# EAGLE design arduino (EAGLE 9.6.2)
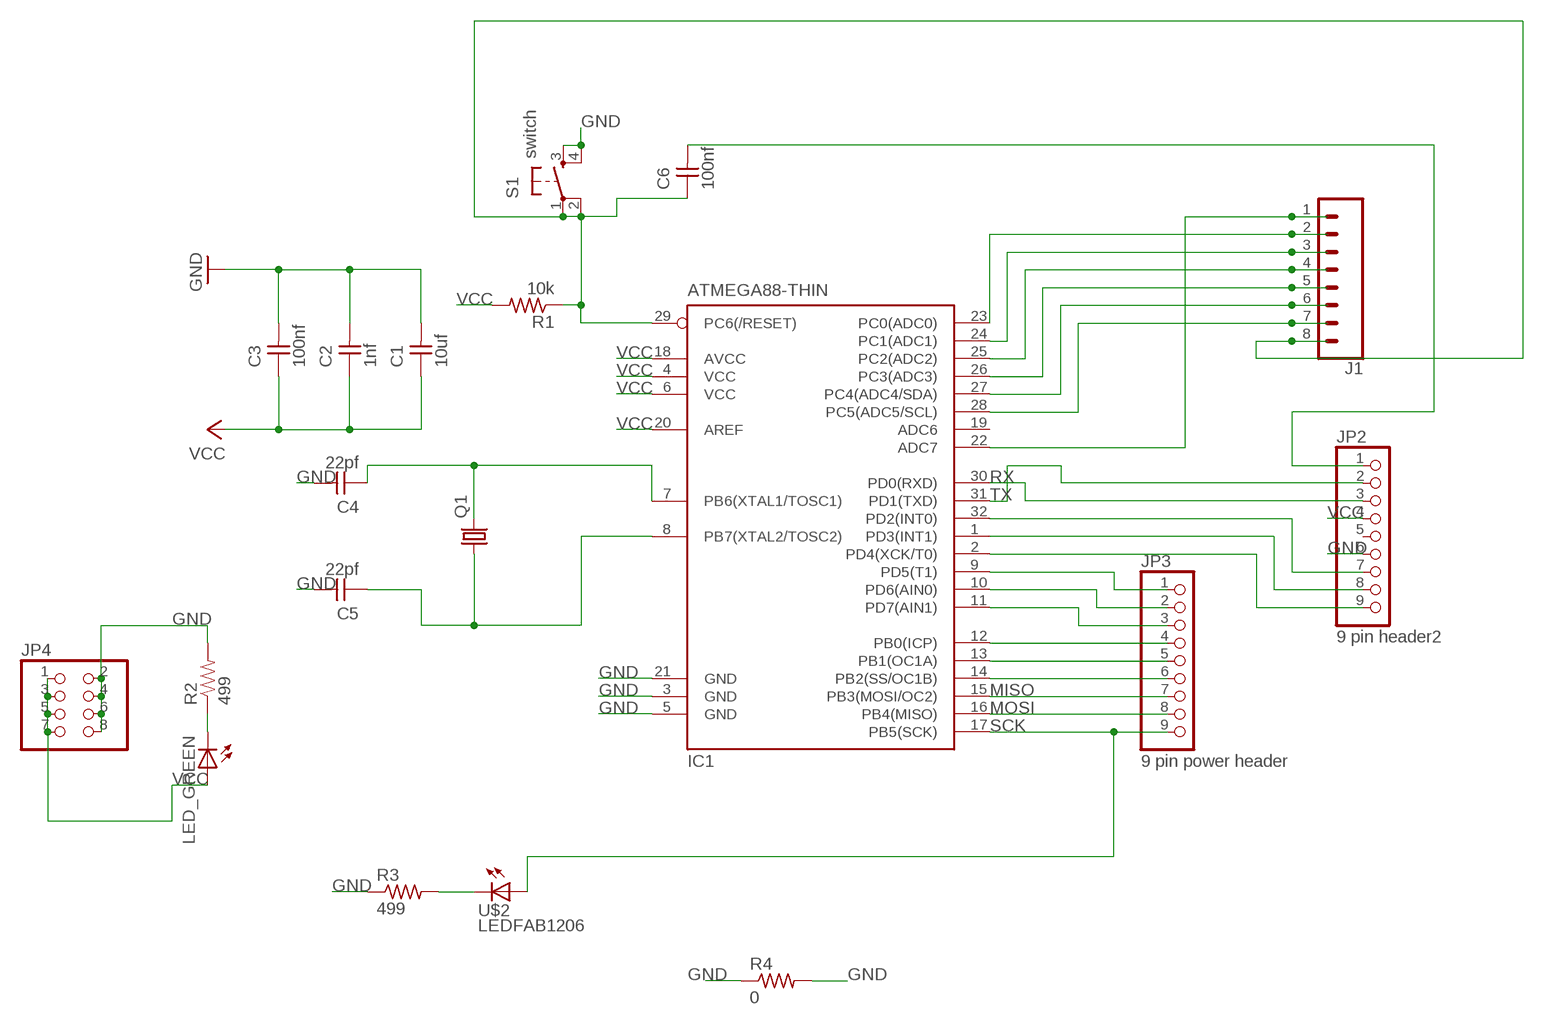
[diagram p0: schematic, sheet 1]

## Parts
C1  10uf  CAP-UNPOLARIZEDFAB  [C1206FAB]
C2  1nf  CAP-UNPOLARIZEDFAB  [C1206FAB]
C3  100nf  CAP-UNPOLARIZEDFAB  [C1206FAB]
C4  22pf  CAP-UNPOLARIZEDFAB  [C1206FAB]
C5  22pf  CAP-UNPOLARIZEDFAB  [C1206FAB]
C6  100nf  CAP-UNPOLARIZEDFAB  [C1206FAB]
IC1  ATMEGA88-THIN  [TQFP32-08THIN]
J1  CONN_08LONGPADS  [1X08_LONGPADS]
JP2  9 pin header2  PINHD-1X9  [1X09]
JP3  9 pin power header  PINHD-1X9  [1X09]
JP4  PINHD-2X4  [2X04]
LED_GREEN  LED1206  [1206]
Q1  CRYSTALHC49S  [HC49/S]
R1  10k  RES-US1206FAB  [R1206FAB]
R2  499  RESISTOR1206  [1206]
R3  499  RES-US1206FAB  [R1206FAB]
R4  0  RES-US1206FAB  [R1206FAB]
S1  switch  6MM_SWITCH6MM_SWITCH  [6MM_SWITCH]
U$2  LEDFAB1206  [LED1206FAB]

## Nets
GND: C1.2 C2.2 C3.2 C4.2 C5.2 IC1.3(GND) IC1.5(GND) IC1.21(GND) JP2.6 JP4.2 JP4.4 JP4.6 JP4.8 R2.2 R3.1 R4.1 R4.2 S1.3(S) S1.4(S1)
MISO: IC1.15(PB3(MOSI/OC2)) JP3.7
MOSI: IC1.16(PB4(MISO)) JP3.8
N$1: IC1.23(PC0(ADC0)) J1.2
N$2: IC1.24(PC1(ADC1)) J1.3
N$3: IC1.25(PC2(ADC2)) J1.4
N$4: IC1.26(PC3(ADC3)) J1.5
N$5: IC1.27(PC4(ADC4/SDA)) J1.6
N$6: IC1.28(PC5(ADC5/SCL)) J1.7
N$7: C6.2 JP2.1
N$8: C6.1 IC1.29(PC6(/RESET)) J1.8 R1.1 S1.1(P) S1.2(P1)
N$9: IC1.22(ADC7) J1.1
N$11: IC1.2(PD4(XCK/T0)) JP2.9
N$12: IC1.1(PD3(INT1)) JP2.8
N$13: IC1.32(PD2(INT0)) JP2.7
N$16: IC1.9(PD5(T1)) JP3.1
N$17: IC1.10(PD6(AIN0)) JP3.2
N$18: IC1.11(PD7(AIN1)) JP3.3
N$19: IC1.12(PB0(ICP)) JP3.4
N$20: IC1.13(PB1(OC1A)) JP3.5
N$21: IC1.14(PB2(SS/OC1B)) JP3.6
N$23: LED_GREEN.2(C) R2.1
N$26: R3.2 U$2.2(C)
N$30: C4.1 IC1.7(PB6(XTAL1/TOSC1)) Q1.2
N$31: C5.1 IC1.8(PB7(XTAL2/TOSC2)) Q1.1
RX: IC1.30(PD0(RXD)) JP2.3
SCK: IC1.17(PB5(SCK)) JP3.9 U$2.1(A)
TX: IC1.31(PD1(TXD)) JP2.2
VCC: C1.1 C2.1 C3.1 IC1.4(VCC) IC1.6(VCC) IC1.18(AVCC) IC1.20(AREF) JP2.4 JP4.1 JP4.3 JP4.5 JP4.7 LED_GREEN.1(A) R1.2
Unconnected: IC1.19(ADC6) JP2.5

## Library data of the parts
C1-C6 = fab:CAP-UNPOLARIZED
IC1 = fab:ATMEGA88-THIN
J1 = SparkFun-Connectors:CONN_08: Multi connection point. Often used as Generic Header-pin footprint for 0.1 inch spaced/style header connections On any of the 0.1 inch spaced packages, you can populate with these: Break Away Headers - Straight (PRT-00116) Break Away Male Headers - Right Angle (PRT-00553) Female Headers (PRT-00115)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
JP2 JP3 = pinhead:PINHD-1X9: PIN HEADER
JP4 = pinhead:PINHD-2X4: PIN HEADER
LED_GREEN = 01_FAB_Hello:LED
Q1 = crystal:CRYSTAL: CRYSTAL; OC_FARNELL: 1667008; OC_NEWARK: unknown
R1 R3 R4 = fab:RES-US: Resistor (US Symbol)
R2 = 01_SparkFun:RESISTOR: Resistor
S1 = fab:6MM_SWITCH: OMRON SWITCH
U$2 = fab:LED: LED

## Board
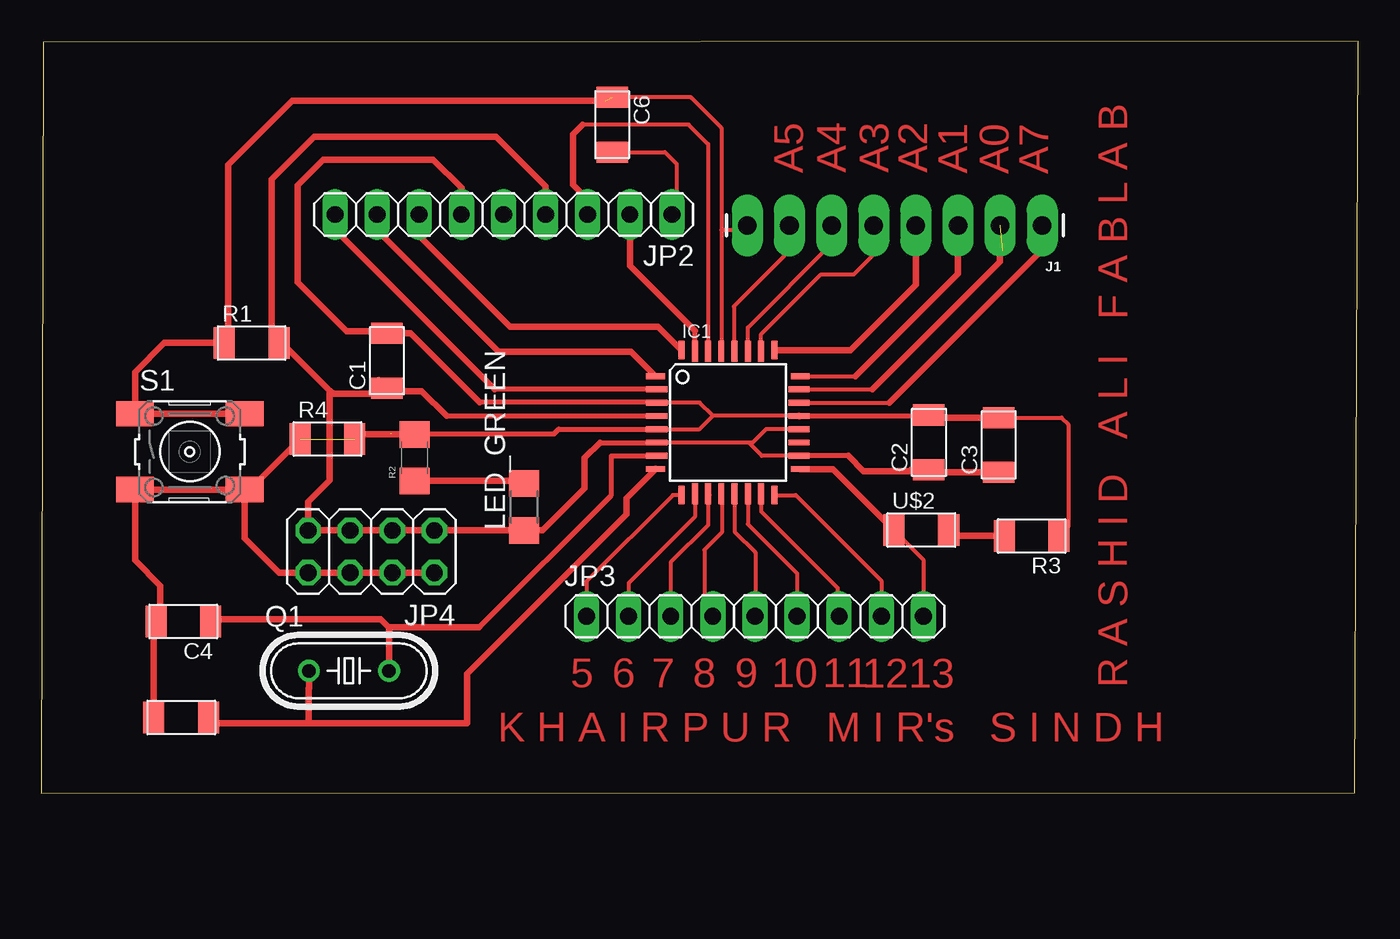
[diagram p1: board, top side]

Size 79.4 x 45.33 mm. Coordinates in mm from the lower left corner, seen from the top.
Outline: 0,0 79.2,0.02 79.4,45.33 0.1,45.28 0,0
Copper layers (1*16): Top 0.035mm / dielectric 1.5mm / Bottom 0.035mm
Design rules "default *": minimum track width 10mil, minimum drill 24mm, track to track 8mil, track to pad 8mil, pad to pad 8mil, via to via 8mil, smd to smd 8mil, copper to edge 40mil, drill to drill 8mil, minimum pad ring 10mil, minimum via ring 8mil, stop-mask expansion 4mil, vias tented up to drill 0mil, thermal gap 10mil

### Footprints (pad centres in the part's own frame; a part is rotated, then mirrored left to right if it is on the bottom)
C1206FAB = smd 1.27 x 1.905: 1 -1.651,0; 2 1.651,0
TQFP32-08THIN = smd 1.118 x 0.356: 1 -4.369,2.8; 8 -4.369,-2.8; 17 4.369,-2.8; 24 4.369,2.8 | smd 1.27 x 0.356: 2 -4.293,2; 3 -4.293,1.2; 4 -4.293,0.4; 5 -4.293,-0.4; 6 -4.293,-1.2; 7 -4.293,-2; 18 4.293,-2; 19 4.293,-1.2; 20 4.293,-0.4; 21 4.293,0.4; 22 4.293,1.2; 23 4.293,2 | smd 0.356 x 1.118: 9 -2.8,-4.369; 16 2.8,-4.369; 25 2.8,4.369; 32 -2.8,4.369 | smd 0.356 x 1.27: 10 -2,-4.293; 14 1.2,-4.293; 15 2,-4.293; 26 2,4.293; 27 1.2,4.293; 31 -2,4.293 | smd 0.35 x 1.27: 11 -1.2,-4.293; 12 -0.4,-4.293; 13 0.4,-4.293; 28 0.4,4.293; 29 -0.4,4.293; 30 -1.2,4.293
1X08_LONGPADS = drill 1.118 pad 1.88 long: 1 0,0; 2 2.54,0; 3 5.08,0; 4 7.62,0; 5 10.16,0; 6 12.7,0; 7 15.24,0; 8 17.78,0
1X09 = drill 1.016 long: 1 -10.16,0; 2 -7.62,0; 3 -5.08,0; 4 -2.54,0; 5 0,0; 6 2.54,0; 7 5.08,0; 8 7.62,0; 9 10.16,0
2X04 = drill 1.016 octagon: 1 -3.81,-1.27; 2 -3.81,1.27; 3 -1.27,-1.27; 4 -1.27,1.27; 5 1.27,-1.27; 6 1.27,1.27; 7 3.81,-1.27; 8 3.81,1.27
1206 = smd 1.6 x 1.803: 1 -1.422,0; 2 1.422,0
HC49/S = drill 0.813: 1 -2.413,0; 2 2.413,0
R1206FAB = smd 1.27 x 1.905: 1 -1.651,0; 2 1.651,0
1206' = smd 1.6 x 1.8: 1 -1.4,0; 2 1.4,0
6MM_SWITCH = smd 2.286 x 1.524: 1 -3.302,2.286; 2 3.302,2.286; 3 -3.302,-2.286; 4 3.302,-2.286
LED1206FAB = smd 1.27 x 1.905: 1 -1.651,0; 2 1.651,0

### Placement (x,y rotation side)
C1  20.83,26.09 90 top
C2  53.52,21.16 90 top
C3  57.73,21.01 90 top
C4  8.56,10.36 180 top
C5  8.43,4.57 180 top
C6  34.42,40.31 270 top
IC1  41.4,22.35 0 top
J1  60.35,34.24 180 top
JP2  27.86,34.9 180 top
JP3  43.03,10.67 0 top
JP4  19.89,14.58 180 top
LED_GREEN  29.11,17.27 90 top
Q1  18.54,7.39 0 top
R1  12.67,27.15 0 top
R2  499  [1206']  22.5,20.24 90 top
R3  59.72,15.52 180 top
R4  17.25,21.36 0 top
S1  8.94,20.6 0 top
U$2  53.06,15.87 0 top

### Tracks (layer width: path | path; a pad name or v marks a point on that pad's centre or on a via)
GND  (2 unrouted)
  Top 0.254: IC1.21 40.49,22.75 | IC1.3 39.69,23.55 40.49,22.75 | 40.49,22.75 39.69,21.95 IC1.5 | C3.2 61.52,22.66 61.92,22.25 61.92,16.08 R3.1
  Top 0.305: 26.43,23.58 37.08,23.58 IC1.3 | 21.08,21.67 30.91,21.67 31.2,21.95 IC1.5 | IC1.21 53.46,22.75 C2.2
  Top 0.406: 45.71,22.73 IC1.21 | C3.2 53.67,22.66 C2.2 | 7.19,4.17 C5.2 6.78,10.24 C4.2 | C4.2 6.91,10.82 | 26.43,23.58 22.28,27.74 C1.2 20.7,27.86 18.39,27.86 15.44,30.81 15.44,36.65 16.99,38.2 23.62,38.2 25.32,36.5 JP2.6 | S1.4 S1.3 5.64,14.05 7.16,12.52 7.16,10.62 C4.2 | JP4.2 JP4.4 JP4.6 JP4.8 14.33,13.31 12.24,15.39 S1.4 | 21.11,21.64 R2.2 19.18,21.64 R4.2 | R4.1 12.55,18.31 S1.4
MISO
  Top 0.254: IC1.15 43.4,17 48.01,12.39 48.01,10.77 JP3.7
MOSI
  Top 0.254: IC1.16 45.49,17.98 50.65,12.83 JP3.8
N$1  (1 unrouted)
  Top 0.254: IC1.23 50.11,24.35
  Top 0.406: 57.81,32.59 57.94,32.72 | 50.11,24.35 57.81,32.06 J1.2
N$2
  Top 0.254: IC1.24 49.1,25.15
  Top 0.406: 49.1,25.15 55.27,31.32 J1.3
N$3
  Top 0.406: IC1.25 48.79,26.72 52.73,30.66 J1.4
N$4
  Top 0.254: IC1.26 43.4,27.68 47.02,31.29 49,31.29 50.19,32.49 J1.5
N$5
  Top 0.254: IC1.27 42.6,28.07 47.65,33.12 J1.6
N$6
  Top 0.254: 41.83,26.67 IC1.28 41.76,26.69 41.76,29.36 45.11,32.72 J1.7
N$7
  Top 0.254: C6.2 37.59,38.66 38.3,37.95 38.3,35.18 JP2.1
N$8  (1 unrouted)
  Top 0.254: 41,33.96 41,40.13 39.17,41.96 C6.1 | 41,33.96 IC1.29 | J1.8 42.29,33.96 41,33.96
  Top 0.406: 34.01,41.76 15.11,41.76 11.25,37.9 11.25,27.84 10.79,27.38 R1.1 7.39,27.15 5.64,25.4 S1.1 S1.2 11.89,22.53
N$9
  Top 0.254: 45.77,23.63 IC1.22 51.14,23.55
  Top 0.406: 51.14,23.55 60.35,32.77 J1.1
N$11
  Top 0.305: IC1.2 27.34,24.35
  Top 0.406: JP2.9 17.76,34.85 17.76,33.93 27.34,24.35
N$12
  Top 0.406: IC1.1 35.56,26.62 27.55,26.62 20.24,33.93 JP2.8
N$13
  Top 0.406: IC1.32 37.18,28.14 28.27,28.14 22.78,33.63 JP2.7
N$16
  Top 0.254: IC1.9 38.08,17.98 32.87,12.78 JP3.1
  Top 0.305: IC1.9
N$17
  Top 0.254: IC1.10 39.4,16.67 35.41,12.68 JP3.2
  Top 0.305: 39.42,18.04 IC1.10
N$18
  Top 0.254: IC1.11 40.2,16.17 37.95,13.92 JP3.3
  Top 0.305: 40.26,18 IC1.11
N$19
  Top 0.254: IC1.12 41.03,18.03 41.03,15.73 39.98,14.68 39.98,11.18 JP3.4
N$20
  Top 0.254: JP3.5 43.05,10.69 43.05,14.53 41.8,15.78 IC1.13
  Top 0.305: 41.83,18.03 IC1.13
N$21
  Top 0.254: IC1.14 42.6,16.22 45.57,13.26 JP3.6
N$23
  Top 0.406: 29.49,19.08 LED_GREEN.2 | LED_GREEN.2 29.03,18.77 | R2.1 28.96,18.84 LED_GREEN.2
N$26
  Top 0.406: R3.2 55.07,15.52 U$2.2
N$30
  Top 0.305: 26.39,10.01 34.37,17.98 34.37,20.35 IC1.7
  Top 0.406: C4.1 10.34,10.49 20.45,10.49 20.95,9.98 Q1.2 20.95,9.88 21.08,10.01 26.39,10.01
N$31
  Top 0.406: IC1.8 35.28,17.8 35.28,16.84 25.65,7.21 25.65,4.24 16.1,4.24 | 10.17,4.48 C5.1 10.41,4.24 16.1,4.24 | Q1.1 16.13,6.35 16.1,6.32 16.1,4.24
RX
  Top 0.254: 32.64,40.31 39.03,40.31 40.2,39.14 IC1.30
  Top 0.406: 32.64,40.31 32.05,39.73 32.05,36.7 32.94,35.81 JP2.3
SCK
  Top 0.254: U$2.1 53.19,14.1 JP3.9
  Top 0.406: U$2.1 47.73,19.55 IC1.17
TX
  Top 0.305: IC1.31 39.4,27.88
  Top 0.406: 39.4,27.88 35.48,31.8 JP2.2
VCC
  Top 0.254: IC1.20 43.69,21.95 42.88,21.13 42.67,21.13 | IC1.6 37.13,21.13 42.67,21.13 | IC1.18 43.45,20.35 42.67,21.13
  Top 0.305: 33.68,21.13 37.13,21.13 | 24.44,22.75 IC1.4 | 48.66,20.35 IC1.18
  Top 0.406: C2.1 52.43,19.51 52.5,19.43 | 52.5,19.43 49.58,19.43 48.66,20.35 | 52.5,19.43 52.58,19.36 C3.1 58.19,19.36 | LED_GREEN.1 30.23,15.85 32.77,18.39 32.77,20.22 33.68,21.13 | C1.1 20.34,24.92 | C1.1 21.01,24.26 22.94,24.26 24.44,22.75 | C1.1 20.83,24.71 | LED_GREEN.1 | LED_GREEN.1 JP4.1 JP4.3 JP4.5 JP4.7 16.08,17.58 17.37,18.87 17.37,24.28 | 17.37,24.28 17.58,24.08 20.47,24.08 C1.1 | 17.37,24.28 14.33,27.33 R1.2 13.87,27.61 13.87,37.01 16.43,39.57 27.43,39.57 30.4,36.6 JP2.4

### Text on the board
Top: R A S H I D A L I F A B L A B | A5 | A4 | A3 | A2 | A1 | A0 | A7 | 5 | 6 | 7 | 8 | 9 | 10 | 11 | 12 | 13 | K H A I R P U R M I R's S I N D H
